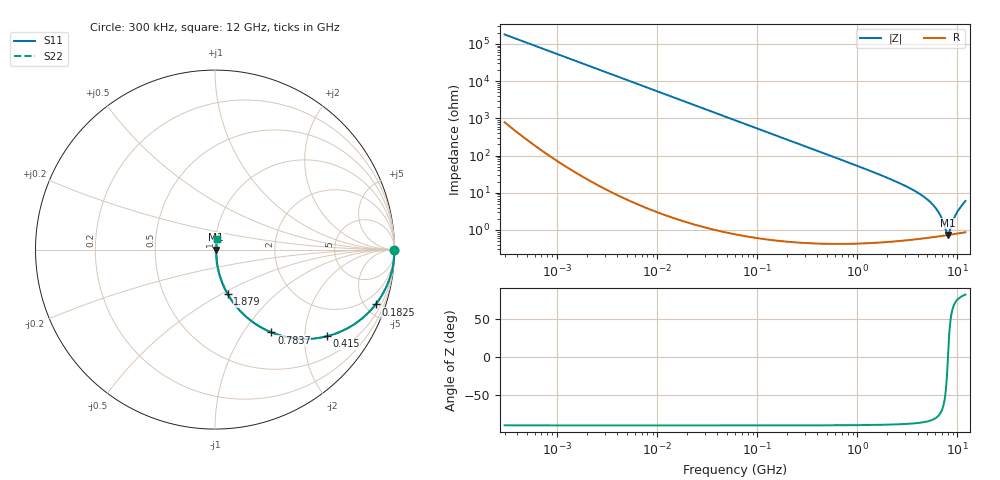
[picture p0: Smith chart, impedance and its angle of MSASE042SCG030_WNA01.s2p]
! MSASE042SCG030_WNA01  S-PARAMETER MODEL  ( General Type )
! Model Generated by TAIYO YUDEN Corporation (http://www.ty-top.com)
! Version 1.0
! TAIYO YUDEN Control No. 130801
! Copyright(c) 2013 TAIYO YUDEN CO.,LTD. All Rights Reserved.
! Product Description (link to TY-COMPAS)
! https://ds.yuden.co.jp/TYCOMPAS/or/detail?pn=MSASE042SCG030AWNA01&u=M
! Products Name : Multilayer Ceramic Capacitors
! Characteristics :
!  Capacitance : 3 pF , Rated Voltage : 16V , TCC : CG / C0G
!  Case Size : 0.4 x 0.2 / 0.016 x 0.008 [mm/inch] , Thickness : 0.2 / 0.008 [mm/inch]
!  (Conditions: Temperature = 25 degC , DC Bias Current/Voltage = 0A / 0V)
! External Node Assignments :
!  1  o---| |---o  2
! GND o---------o GND
! Frequency Range : 0.3MHz  -  12000MHz  [ 401 STEP ]
# MHz S RI R 50
! Freq[MHz].  S11 Real  S11 Imag  S21 Real  S21 Imag  S12 Real  S12 Imag  S22 Real  S22 Imag
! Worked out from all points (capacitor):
!   401 points, 300 kHz to 12 GHz, reference 50 ohm
!   read as one part in series: C = 2.98 pF near 316.3 kHz
!   lowest |Z| = 733 mohm at 8.065 GHz (marker M1)
!   series resonance near 8.045 GHz, so ESL is about 130 pH
!   S11 on the Smith chart (normalised r, x): 300 kHz: open; 182.5 MHz: 1.01, -5.86; 415 MHz: 1.01, -2.57; 783.7 MHz: 1.01, -1.35; 1.879 GHz: 1.01, -0.54; 12 GHz: 1.02, +0.12
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0.3  1 -0.000561  2.77e-06 0.000561  2.77e-06 0.000561  1 -0.000561
1.769972  1 -0.00331  1.4e-05 0.00331  1.4e-05 0.00331  1 -0.00331
10.44266  0.9996 -0.0195  0.000392 0.0195  0.000392 0.0195  0.9996 -0.0195
60  0.9875 -0.1108  0.0125 0.1108  0.0125 0.1108  0.9875 -0.1108
182.544  0.8951 -0.3055  0.1049 0.3055  0.1049 0.3055  0.8951 -0.3055
353.9943  0.694 -0.4594  0.306 0.4594  0.306 0.4594  0.694 -0.4594
414.98  0.6225 -0.4831  0.3775 0.4831  0.3775 0.4831  0.6225 -0.4831
570.2811  0.4655 -0.4965  0.5345 0.4965  0.5345 0.4965  0.4655 -0.4965
783.7017  0.3147 -0.4613  0.6853 0.4613  0.6853 0.4613  0.3147 -0.4613
1197.383  0.1627 -0.3641  0.8373 0.3641  0.8373 0.3641  0.1627 -0.3641
1878.541  0.0713 -0.2488  0.9287 0.2488  0.9287 0.2488  0.0713 -0.2488
2088.533  0.058 -0.2239  0.942 0.2239  0.942 0.2239  0.058 -0.2239
3642.919  0.0187 -0.114  0.9813 0.114  0.9813 0.114  0.0187 -0.114
5278.635  0.00947 -0.057  0.9905 0.057  0.9905 0.057  0.00947 -0.057
6524.734  0.00747 -0.0278  0.9925 0.0278  0.9925 0.0278  0.00747 -0.0278
7064.448  0.00719 -0.0173  0.9928 0.0173  0.9928 0.0173  0.00719 -0.0173
7648.807  0.00716 -0.00685  0.9928 0.00685  0.9928 0.00685  0.00716 -0.00685
8064.993  0.00726 0.000359  0.9927 -0.000359  0.9927 -0.000359  0.00726 0.000359
8503.825  0.00749 0.00798  0.9925 -0.00798  0.9925 -0.00798  0.00749 0.00798
9207.246  0.00801 0.0185  0.992 -0.0185  0.992 -0.0185  0.00801 0.0185
9968.853  0.0088 0.0293  0.9912 -0.0293  0.9912 -0.0293  0.0088 0.0293
12000  0.012 0.0583  0.988 -0.0583  0.988 -0.0583  0.012 0.0583
